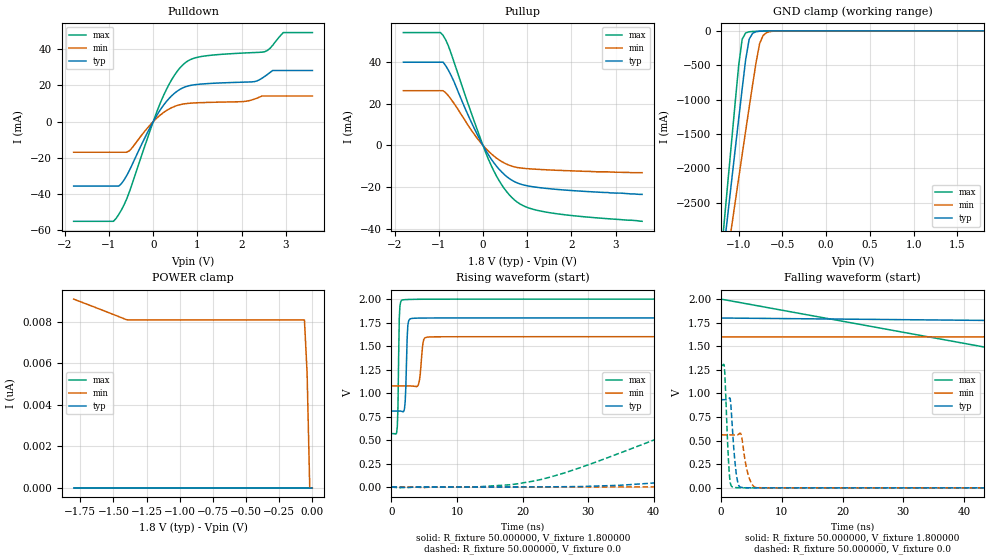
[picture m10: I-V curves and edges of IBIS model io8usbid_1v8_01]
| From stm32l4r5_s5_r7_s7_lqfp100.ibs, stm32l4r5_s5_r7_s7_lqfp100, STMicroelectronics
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|   Model io8usbid_1v8_01
[Model]  io8usbid_1v8_01
Model_type I/O
Polarity   Non-Inverting
Enable   Active-Low
Vinl =   0.540000V
Vinh =   1.260000V
Vmeas =  0.900000V
Cref =   100.000000nF
Rref =   1.000000k
Vref =   1.800000V
C_comp   2.022300pF   2.021100pF   2.049600pF
[Temperature Range]   25.000000   0.125000k   -40.000000
[Pullup Reference]   1.800000V   1.600000V   2.000000V
[Pulldown Reference]   0.0V   0.0V   0.0V
[POWER Clamp Reference]   1.800000V   1.600000V   2.000000V
[GND Clamp Reference]   0.0V   0.0V   0.0V
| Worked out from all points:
|   slope of the pulldown table from 0 to 0.27 V, typ, clamps not added: 26.4 ohm
|   slope of the pullup table from 0 to 0.27 V, typ, clamps not added: 30.1 ohm
|   GND clamp passes 1 mA (typ) near -0.60 V on its own axis
|   rising waveform, R_fixture 50.000000, V_fixture 1.800000: 20-80 % time 251ps typ, 397ps min, 180ps max; typ from 0.809 V to 1.8 V
|   rising waveform, R_fixture 50.000000, V_fixture 0.0: 20-80 % time 65ns typ, 114ns min, 35.5ns max; typ from 0 V to 0.934 V
|   falling waveform, R_fixture 50.000000, V_fixture 1.800000: 20-80 % time 75.9ns typ, 121ns min, 62.9ns max; typ from 1.8 V to 0.809 V
|   falling waveform, R_fixture 50.000000, V_fixture 0.0: 20-80 % time 682ps typ, 987ps min, 518ps max; typ from 0.934 V to 0 V
[Pulldown]
|Voltage   I(typ)   I(min)   I(max)
-1.8V     -35.64mA   -16.93mA   -55.1mA
-840mV    -35.64mA   -16.93mA   -53.52mA
-720mV    -34.31mA   -16.93mA   -48.86mA
-540mV    -27.04mA   -16.13mA   -38.89mA
240mV     9.303mA    5.14mA     14.78mA
480mV     15.67mA    8.374mA    25.64mA
720mV     19.18mA    9.883mA    32.46mA
1.14V     20.87mA    10.54mA    36.19mA
2.28V     22.08mA    12.35mA    38.18mA
2.52V     24.96mA    14.16mA    38.63mA
2.94V     28.27mA    14.16mA    49.23mA
3.6V      28.27mA    14.16mA    49.23mA
[Pullup]
|Voltage   I(typ)   I(min)   I(max)
-1.8V     39.84mA    26.17mA    54.03mA
-960mV    39.84mA    26.17mA    54.03mA
-900mV    39.84mA    26.17mA    52.65mA
-780mV    35.95mA    23.7mA     47.58mA
-240mV    10.08mA    6.588mA    14.1mA
120mV     -4.38mA    -2.702mA   -6.45mA
240mV     -8.143mA   -5.004mA   -12mA
420mV     -12.68mA   -7.723mA   -18.77mA
720mV     -17.48mA   -10.37mA   -26.28mA
1.02V     -19.45mA   -11.2mA    -29.89mA
1.5V      -20.78mA   -11.79mA   -32.25mA
3.6V      -23.5mA    -13.1mA    -36.4mA
[GND_clamp]
|Voltage   I(typ)   I(min)   I(max)
-1.8V     -9.895A    -9.296A    -9.457A
-1.2V     -3.533A    -3.902A    -3.274A
-1.16V    -3.082A    -3.55A     -2.716A
-1.12V    -2.631A    -3.198A    -2.159A
-1.08V    -2.182A    -2.848A    -1.604A
-1V       -1.289A    -2.15A     -512mA
-960mV    -849.4mA   -1.803A    -123.8mA
-920mV    -422.4mA   -1.459A    -30.79mA
-880mV    -123.7mA   -1.118A    -13.63mA
-760mV    -6.32mA    -185mA     -5.692mA
-680mV    -2.569mA   -25.43mA   -2.907mA
1.8V      0A         0A         0A
[POWER_clamp]
|Voltage   I(typ)   I(min)   I(max)
-1.8V     0A         9.088nA    0A
-1.4V     0A         8.095nA    0A
-60mV     0A         8.084nA    0A
-40mV     0A         5.54nA     0A
-20mV     0A         0A         0A
0V        0A         0A         0A
[Ramp]
| variable   typ   min   max
dV/dt_r  0.56065/64.96581n   0.33685/0.11408u   0.77868/35.44838n
dV/dt_f  0.59474/66.70595n   0.31470/0.11610u   0.85906/34.89439n
R_load = 50.000000
[Rising Waveform]
R_fixture= 50.000000
V_fixture= 1.800000
V_fixture_min= 1.600000
V_fixture_max= 2.000000
|time   V(typ)   V(min)   V(max)
0s        808.7mV    1.076V     568.3mV
900.9ps   808.8mV    1.076V     643.9mV
1.201ns   808.7mV    1.076V     1.796V
1.602ns   805mV      1.076V     1.989V
2.102ns   909.9mV    1.076V     1.995V
2.503ns   1.717V     1.076V     1.996V
3.003ns   1.793V     1.075V     1.997V
4.104ns   1.798V     1.087V     1.998V
5.506ns   1.799V     1.595V     1.999V
49.85ns   1.8V       1.6V       2V
[Rising Waveform]
R_fixture= 50.000000
V_fixture= 0.0
V_fixture_min= 0.0
V_fixture_max= 0.0
|time   V(typ)   V(min)   V(max)
0s        740.2nV    986nV      -25.48nV
13.21ns   -57.76uV   -37.13uV   2.605mV
22.82ns   1.56mV     -18.62uV   80.34mV
50.45ns   121.4mV    4.939mV    756.2mV
68.47ns   310.5mV    20.98mV    1.064V
82.88ns   461.2mV    49.95mV    1.188V
102.1ns   629mV      109.3mV    1.253V
161ns     870.8mV    314.5mV    1.294V
253.5ns   929.1mV    496.9mV    1.298V
598.2ns   934.4mV    561.5mV    1.298V
[Falling Waveform]
R_fixture= 50.000000
V_fixture= 1.800000
V_fixture_min= 1.600000
V_fixture_max= 2.000000
|time   V(typ)   V(min)   V(max)
0s        1.8V       1.6V       2V
50.05ns   1.77V      1.6V       1.414V
100.1ns   1.343V     1.568V     664.1mV
150.2ns   974mV      1.436V     590.2mV
200.2ns   869mV      1.276V     574.5mV
250.2ns   834.2mV    1.178V     569.8mV
300.3ns   820.1mV    1.132V     568.8mV
400.4ns   810.6mV    1.095V     568.3mV
500.5ns   809.2mV    1.082V     568.3mV
4.955us   808.7mV    1.076V     568.3mV
[Falling Waveform]
R_fixture= 50.000000
V_fixture= 0.0
V_fixture_min= 0.0
V_fixture_max= 0.0
|time   V(typ)   V(min)   V(max)
0s        934.4mV    561.5mV    1.298V
500.5ps   934.4mV    561.5mV    1.304V
1.301ns   945.9mV    561.5mV    194mV
1.502ns   942.7mV    561.5mV    55.41mV
1.902ns   586.5mV    561.4mV    8.471mV
2.503ns   145.6mV    560.8mV    2.359mV
3.303ns   5.348mV    564.8mV    1.106mV
4.404ns   832.5uV    151.6mV    678.6uV
5.706ns   250.4uV    4.111mV    436.1uV
49.85ns   740.2nV    986nV      -25.48nV
